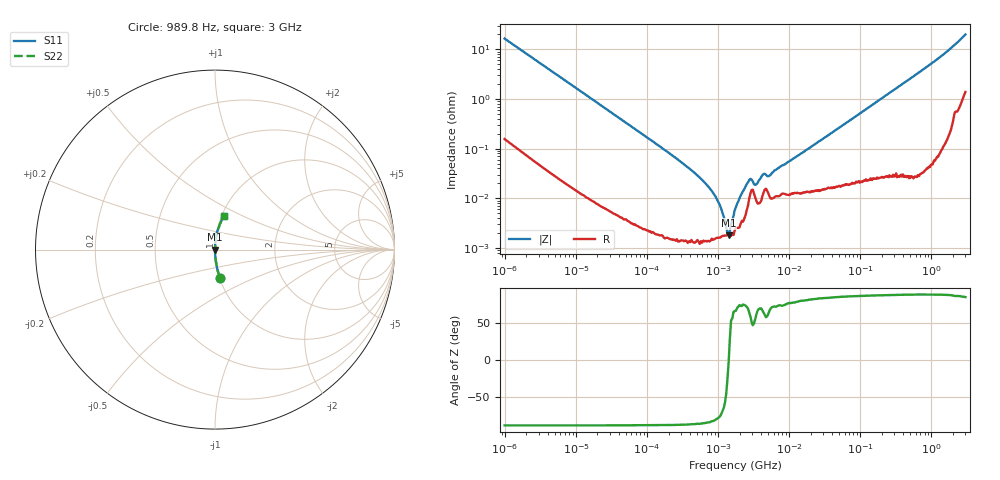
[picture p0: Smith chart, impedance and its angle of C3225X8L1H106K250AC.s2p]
! S-Parameter Data Generated by TDK Corporation
! Copyright(C) 2024 TDK Corporation.
! All Rights Reserved.
! TDK P/N: C3225X8L1H106K250AC (Multilayer Ceramic Chip Capacitor)
! Property: C=10uF
! Size(LxWxT): 3.2x2.5x2.5mm
! Model Type: s2p (Touchstone File Format Version 1.0)
! Frequency: DC=Yes Start=0.000989846MHz Stop=3000MHz 523points Log-sweep
! Model Generated on May 28, 2024
! Terms and conditions regarding TDK Simulation Models:
! 1)This simulation model is being provided solely for informational
!  purposes. Please refer to the specifications of the products in
!  terms of detailed characteristics of such products.
! 2)In no event shall TDK Corporation of any of its subsidiaries be
!  liable for any loss or damage arising, directly or indirectly,
!  from any information contained in this simulation model, including,
!  but not limited to loss or damages arising from any inaccuracies,
!  omissions or errors in connection with such information.
! 3)Any and all copyrights on this simulation model are owned by
!  TDK Corporation.  Duplication or redistribution of this simulation
!  model without prior written permission from TDK Corporation
!  is prohibited.
! 4)This simulation model is subject to any modification or change
!  without any prior notice.
! 5)Neither TDK Corporation nor any of its subsidiaries shall make any
!  warranty, express or implied, including but not limited to the
!  correctness, implied warranties of merchantability and fitness for
!  a particular purpose with respect to this simulation models.
! 6)The use of this simulation model shall be deemed to have consented
!  to the terms and conditions hereof.
! Port Assignments:
!  1 ---| |--- 2
! Applicable Conditions:
!  Temperature = 25 degC
!  DC Bias Voltage = 0 V
!  Small Signal Operation
# Hz S MA R 50
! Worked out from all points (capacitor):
!   522 points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, 989.8 Hz to 3 GHz, reference 50 ohm
!   read as one part in series: C = 9.73 uF near 1.07 kHz
!   lowest |Z| = 1.81 mohm at 1.404 MHz (marker M1)
!   series resonance near 1.408 MHz, so ESL is about 1.3 nH
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989.846  0.1622 -80.1  0.9852 9.3  0.9852 9.3  0.1622 -80.1
2838.53  0.05797 -86.2  0.9978 3.3  0.9978 3.3  0.05797 -86.2
12024.6  0.01387 -88.7  0.9998 0.8  0.9998 0.8  0.01387 -88.7
146075  0.001146 -89.0  1 0.1  1 0.1  0.001146 -89.0
470910  0.0003196 -87.7  1 0.0  1 0.0  0.0003196 -87.7
669031  0.0001963 -86.0  1 0.0  1 0.0  0.0001963 -86.0
950505  9.778e-05 -80.6  1 0.0  1 0.0  9.778e-05 -80.6
1027650  7.885e-05 -78.2  1 0.0  1 0.0  7.885e-05 -78.2
1404130  1.805e-05 -2.3  1 0.0  1 0.0  1.805e-05 -2.3
1774520  6.586e-05 67.3  1 -0.0  1 -0.0  6.586e-05 67.3
1918540  8.698e-05 73.1  1 -0.0  1 -0.0  8.698e-05 73.1
2074250  0.000113 74.1  1 -0.0  1 -0.0  0.000113 74.1
2725710  0.0002324 65.2  0.9999 -0.0  0.9999 -0.0  0.0002324 65.2
2946930  0.0002388 52.1  0.9999 -0.0  0.9999 -0.0  0.0002388 52.1
3444700  0.0001905 62.3  0.9999 -0.0  0.9999 -0.0  0.0001905 62.3
4353360  0.0003081 64.6  0.9999 -0.0  0.9999 -0.0  0.0003081 64.6
5291160  0.0002859 67.9  0.9999 -0.0  0.9999 -0.0  0.0002859 67.9
7229600  0.0004173 74.7  0.9999 -0.0  0.9999 -0.0  0.0004173 74.7
2.09559e7  0.001127 82.9  0.9999 -0.1  0.9999 -0.1  0.001127 82.9
2.50734e8  0.01285 88.1  0.9997 -0.7  0.9997 -0.7  0.01285 88.1
1.21884e9  0.06384 85.7  0.9973 -3.7  0.9973 -3.7  0.06384 85.7
3e9  0.1932 74.9  0.9678 -11.1  0.9678 -11.1  0.1932 74.9
